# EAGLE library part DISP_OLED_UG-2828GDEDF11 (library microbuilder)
128x128 1.5" RGB OLED - UG-2828GDEDF11 30-Pin 0.5mm Pitch FPC Cable (Top+Bottom Contacts) - OMRON XF2M-3015-1A (Digikey: OR723TR-ND) This FPC connector has contacts on the top and bottom, but the appropriate pin needs to be selected depending on whether the OLED will be inserted right-side up (use the TOP pinout) or upside-down (use the BOTTOM pinout).
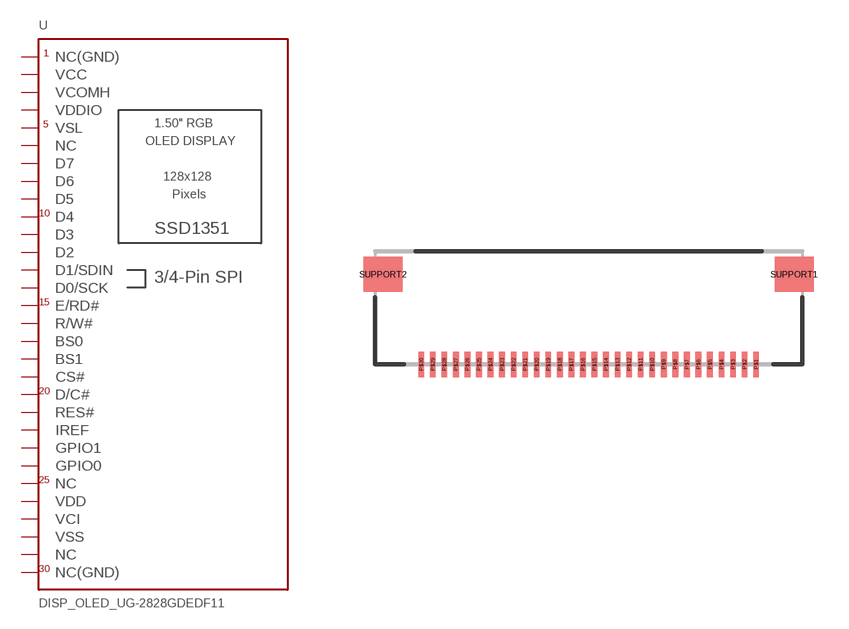
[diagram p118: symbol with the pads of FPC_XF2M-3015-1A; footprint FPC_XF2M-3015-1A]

Designator prefix U

## DISP_OLED_UG-2828GDEDF11TOP  [FPC_XF2M-3015-1A]
P$1  NC(GND)  nc
P$2  NC  nc
P$3  VSS  pwr
P$4  VCI  pwr
P$5  VDD  pwr
P$6  NC  nc
P$7  GPIO0
P$8  GPIO1
P$9  IREF
P$10  RES#
P$11  D/C#
P$12  CS#
P$13  BS1
P$14  BS0
P$15  R/W#
P$16  E/RD#
P$17  D0/SCK
P$18  D1/SDIN
P$19  D2
P$20  D3
P$21  D4
P$22  D5
P$23  D6
P$24  D7
P$25  NC  nc
P$26  VSL
P$27  VDDIO  pwr
P$28  VCOMH  pwr
P$29  VCC  pwr
P$30  NC(GND)  nc

## DISP_OLED_UG-2828GDEDF11BOTTOM  [FPC_XF2M-3015-1A]
P$1  NC(GND)  nc
P$2  VCC  pwr
P$3  VCOMH  pwr
P$4  VDDIO  pwr
P$5  VSL
P$6  NC  nc
P$7  D7
P$8  D6
P$9  D5
P$10  D4
P$11  D3
P$12  D2
P$13  D1/SDIN
P$14  D0/SCK
P$15  E/RD#
P$16  R/W#
P$17  BS0
P$18  BS1
P$19  CS#
P$20  D/C#
P$21  RES#
P$22  IREF
P$23  GPIO1
P$24  GPIO0
P$25  NC  nc
P$26  VDD  pwr
P$27  VCI  pwr
P$28  VSS  pwr
P$29  NC  nc
P$30  NC(GND)  nc

## Footprint FPC_XF2M-3015-1A (pad centres in mm)
30-Pin 0.5mm FPC Top+Bottom - OMRON - XF2M-3015-1A
smd 0.25 x 1.1: P$1 7.25,-2.63; P$2 6.75,-2.63; P$3 6.25,-2.63; P$4 5.75,-2.63; P$5 5.25,-2.63; P$6 4.75,-2.63; P$7 4.25,-2.63; P$8 3.75,-2.63; P$9 3.25,-2.63; P$10 2.75,-2.63; P$11 2.25,-2.63; P$12 1.75,-2.63; P$13 1.25,-2.63; P$14 0.75,-2.63; P$15 0.25,-2.63; P$16 -0.25,-2.63; P$17 -0.75,-2.63; P$18 -1.25,-2.63; P$19 -1.75,-2.63; P$20 -2.25,-2.63; P$21 -2.75,-2.63; P$22 -3.25,-2.63; P$23 -3.75,-2.63; P$24 -4.25,-2.63; P$25 -4.75,-2.63; P$26 -5.25,-2.63; P$27 -5.75,-2.63; P$28 -6.25,-2.63; P$29 -6.75,-2.63; P$30 -7.25,-2.63
smd 1.7 x 1.5: SUPPORT1 8.9,1.27; SUPPORT2 -8.9,1.27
